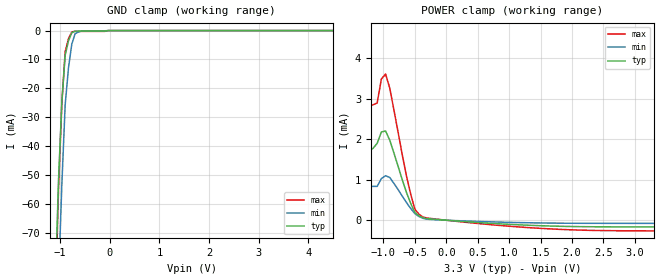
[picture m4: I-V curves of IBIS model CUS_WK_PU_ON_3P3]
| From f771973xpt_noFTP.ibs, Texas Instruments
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|   Model Cell CUS_WK_PU_ON_3P3
|CUS_WK_PU_ON_3P3
[Model]   CUS_WK_PU_ON_3P3
Model_type   Input
Polarity   Non-Inverting
Vinl =  0.8
Vinh =  2
C_comp   2.12034p   1.0392p   2.53442p
[Model Spec]
Vinl   0.8   0.8   0.8
Vinh   2   2   2
[Temperature Range]   25   155   -40
[Voltage Range]   3.3   2.97   3.63
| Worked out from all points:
|   GND clamp passes 1 mA (typ) near -0.77 V on its own axis
|   POWER clamp passes 1 mA (typ) near -0.70 V on its own axis
| Nom Voltages:
|   BIASFET=3.3, VDD=1.2, VDDS=3.3, VSS=0
| Min Voltages:
|   BIASFET=2.97, VDD=1.08, VDDS=2.97, VSS=0
| Max Voltages:
|   BIASFET=3.63, VDD=1.32, VDDS=3.63, VSS=0
[POWER_clamp]
|   voltage   I(typ)   I(min)   I(max)
-3.3V     2.123mA    637.3mA    3.592mA
-2.167V   1.755mA    7.137mA    2.972mA
-2.1V     1.749mA    1.704mA    2.953mA
-1.967V   1.738mA    883.5uA    2.921mA
-1.167V   1.771mA    834.5uA    2.844mA
-1.1V     1.897mA    834.3uA    2.891mA
-1.033V   2.175mA    1.026mA    3.482mA
-966.7mV  2.2mA      1.099mA    3.603mA
-566.7mV  413.8uA    290uA      640.9uA
-500mV    187.7uA    161.3uA    268uA
-366.7mV  54.9uA     44.56uA    74.4uA
3.3V      -165.3uA   -77.84uA   -262.4uA
[GND_clamp]
|   voltage   I(typ)   I(min)   I(max)
-3.3V     -2.204A    -1.834A    -3.186A
-1.1V     -88.86mA   -124.4mA   -95.56mA
-1.033V   -51.39mA   -86.07mA   -54.53mA
-966.7mV  -24.62mA   -53.17mA   -25.11mA
-900mV    -8.575mA   -25.73mA   -7.315mA
-833.3mV  -3.567mA   -12.91mA   -2.804mA
-766.7mV  -776.7uA   -4.697mA   -455.7uA
-700mV    -205.1uA   -1.081mA   -268.8uA
-566.7mV  -167.2uA   -156.8uA   -264.7uA
-500mV    -166.3uA   -89.09uA   -264.6uA
-33.33mV  0A         0A         0A
6.6V      0A         0A         0A
